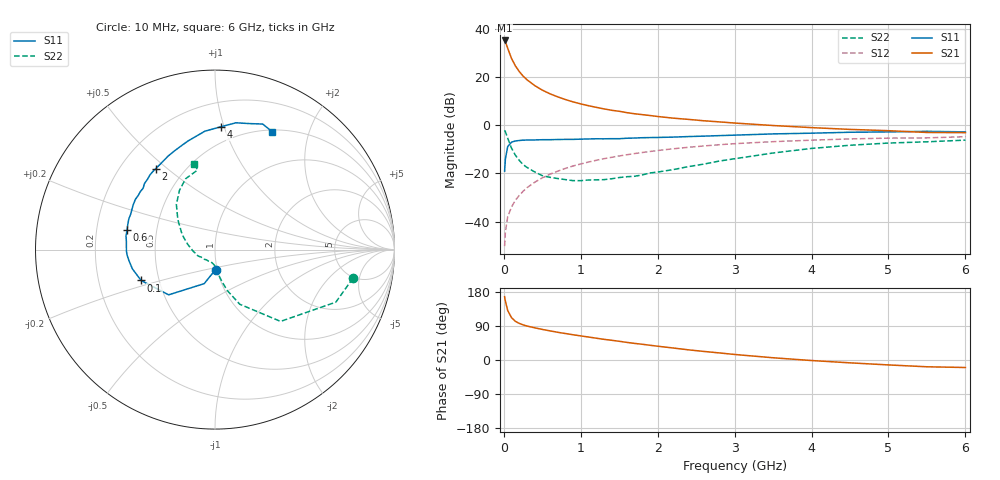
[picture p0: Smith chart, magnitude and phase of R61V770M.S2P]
! SIEMENS Small Signal Semiconductors
! BFR193
! Si NPN RF Bipolar Junction Transistor in SOT23
! VCE = 1.75 V  IC = 70 mA
! Common Emitter S-Parameters:  May  1996
# GHz  S  MA  R  50
!  f  S11  S21  S12  S22
! GHz  MAG  ANG  MAG  ANG  MAG  ANG  MAG  ANG
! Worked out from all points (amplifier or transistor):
!   36 points, 10 MHz to 6 GHz, reference 50 ohm
!   highest |S21| = 35.2 dB at 10 MHz (marker M1)
!   |S21| within 3 dB of that: start of sweep to 47.72 MHz
!   unconditionally stable (mu >= 1): start of sweep to 11.08 MHz; 209.4 MHz to 2.288 GHz
!   at 250 MHz: K = 1.02, MAG = 23.0 dB, |S12| = -27.4 dB
!   at 1.4 GHz: K = 1.04, MAG = 8.5 dB, |S12| = -13.3 dB
!   at 6 GHz: K = 0.99, MSG = 0.8 dB, |S12| = -4.7 dB
!   S11 on the Smith chart (normalised r, x): 10 MHz: 0.98, -0.22; 100 MHz: 0.40, -0.17; 600 MHz: 0.34, +0.10; 2 GHz: 0.35, +0.46; 4 GHz: 0.38, +0.97; 6 GHz: 0.52, +1.47
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0.01  0.1114 -88.4  57.52 167.1  0.0031 77.0  0.785 -11.7
0.02  0.199 -107.6  53.95 155.4  0.0061 72.6  0.7342 -23.5
0.05  0.3608 -135.7  39.8 130.7  0.0126 68.0  0.5417 -47.6
0.1  0.4461 -157.3  24.34 111.6  0.0202 70.6  0.3344 -65.6
0.15  0.4726 -166.9  17.08 102.1  0.0278 71.8  0.2392 -73.2
0.2  0.4831 -172.6  13.05 96.6  0.0349 73.8  0.1871 -77.3
0.25  0.4912 -176.7  10.49 92.7  0.0426 74.6  0.1529 -80.6
0.3  0.4936 -179.4  8.824 89.7  0.0505 75.1  0.1338 -82.6
0.4  0.4956 174.9  6.686 85.0  0.0655 74.9  0.1079 -86.5
0.5  0.5017 171.2  5.362 80.7  0.0811 74.5  0.0901 -90.6
0.6  0.5018 167.5  4.496 76.9  0.0965 73.7  0.0831 -94.6
0.8  0.5097 160.3  3.421 69.9  0.1273 71.1  0.0746 -103.8
0.9  0.5096 157.0  3.057 66.6  0.1429 69.8  0.071 -108.9
1.1  0.5199 151.0  2.547 60.6  0.1727 66.8  0.0732 -119.4
1.6  0.5383 136.9  1.827 46.4  0.2448 58.8  0.0856 -146.5
2  0.5586 126.4  1.521 36.4  0.2991 52.2  0.107 -166.7
2.2  0.5681 121.5  1.407 31.7  0.3249 48.9  0.1202 -174.6
3.5  0.662 94.9  0.988 5.9  0.4571 27.0  0.266 141.1
4  0.6851 87.3  0.894 -1.4  0.4906 19.8  0.3307 130.6
4.5  0.7162 80.6  0.821 -7.5  0.5206 12.7  0.3852 120.9
5.5  0.7484 69.2  0.709 -17.9  0.5478 -0.8  0.454 102.3
6  0.7297 64.0  0.703 -19.8  0.5791 -4.8  0.4913 103.7
